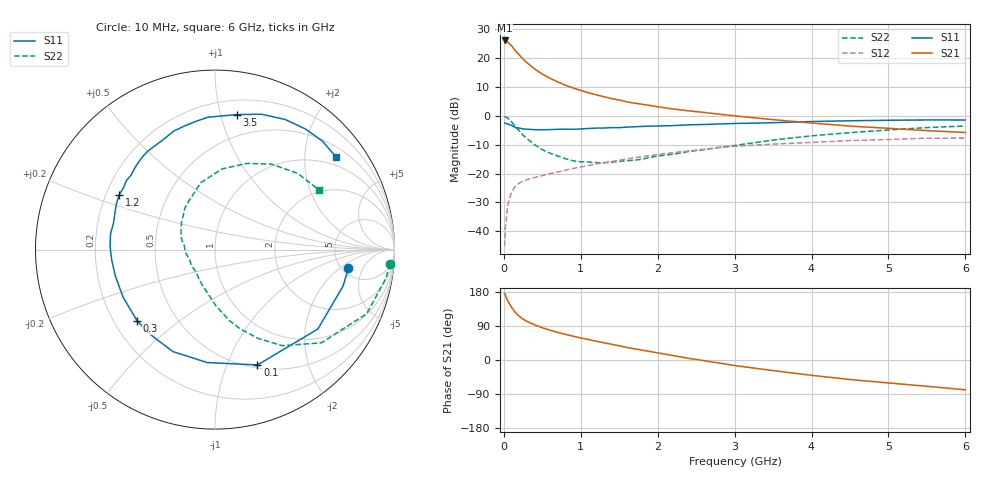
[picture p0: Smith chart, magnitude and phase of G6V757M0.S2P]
! SIEMENS Small Signal Semiconductors
! BFG193
! Si NPN RF Bipolar Junction Transistor in SOT223
! VCE = 0.75 V  IC = 7 mA
! Common Emitter S-Parameters:  August  1996
# GHz  S  MA  R  50
!  f  S11  S21  S12  S22
! GHz  MAG  ANG  MAG  ANG  MAG  ANG  MAG  ANG
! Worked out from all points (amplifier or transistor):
!   36 points, 10 MHz to 6 GHz, reference 50 ohm
!   highest |S21| = 26.2 dB at 10 MHz (marker M1)
!   |S21| within 3 dB of that: start of sweep to 133.7 MHz
!   unconditionally stable (mu >= 1): 910.3 MHz to 3.813 GHz
!   at 250 MHz: K = 0.44, MSG = 21.2 dB, |S12| = -22.6 dB
!   at 1.4 GHz: K = 1.10, MAG = 9.0 dB, |S12| = -15.8 dB
!   at 6 GHz: K = 0.98, MSG = 1.0 dB, |S12| = -7.7 dB
!   S11 on the Smith chart (normalised r, x): 10 MHz: 5.74, -2.68; 100 MHz: 0.53, -1.29; 300 MHz: 0.30, -0.36; 1.2 GHz: 0.25, +0.25; 3.5 GHz: 0.31, +1.13; 6 GHz: 0.75, +2.77
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0.01  0.7507 -7.8  20.35 175.1  0.0055 86.8  0.9785 -4.7
0.02  0.7419 -15.9  20.14 171.1  0.0114 85.6  0.9663 -9.4
0.05  0.724 -37.7  19.13 156.6  0.0278 72.4  0.9178 -22.9
0.1  0.6848 -69.8  16.43 139.4  0.0482 59.5  0.7885 -41.2
0.15  0.6308 -93.9  13.51 125.0  0.0603 49.1  0.6533 -55.0
0.2  0.6148 -112.4  11.43 115.6  0.0681 44.7  0.5492 -64.2
0.25  0.5947 -126.5  9.675 107.8  0.074 41.1  0.4629 -72.4
0.3  0.5883 -137.4  8.36 101.9  0.0783 39.4  0.4047 -78.4
0.4  0.5768 -152.6  6.525 92.9  0.0856 37.7  0.3161 -88.7
0.5  0.5743 -165.3  5.304 85.1  0.0922 36.9  0.2593 -97.1
0.6  0.5783 -174.1  4.49 78.7  0.0997 37.1  0.2252 -104.8
0.8  0.5887 171.4  3.402 67.7  0.1143 37.1  0.1812 -120.9
0.9  0.5844 165.5  3.053 62.8  0.1228 37.2  0.1663 -128.2
1.1  0.6048 155.5  2.52 54.0  0.1378 36.7  0.1582 -144.1
1.2  0.615 150.5  2.327 49.7  0.1461 36.0  0.1547 -151.9
1.6  0.6381 134.3  1.752 33.2  0.1798 31.4  0.167 -178.5
2.2  0.6786 114.8  1.319 11.7  0.2307 21.7  0.2165 150.9
2.8  0.7238 97.9  1.071 -8.1  0.2816 10.0  0.2856 126.1
3.5  0.7621 80.8  0.86 -28.0  0.3243 -6.1  0.3813 102.0
4.5  0.8234 61.7  0.666 -51.6  0.3737 -25.0  0.5118 69.7
5.5  0.8507 45.3  0.556 -69.4  0.4115 -47.5  0.6269 42.6
6  0.849 37.4  0.515 -78.7  0.412 -60.3  0.6683 29.8
